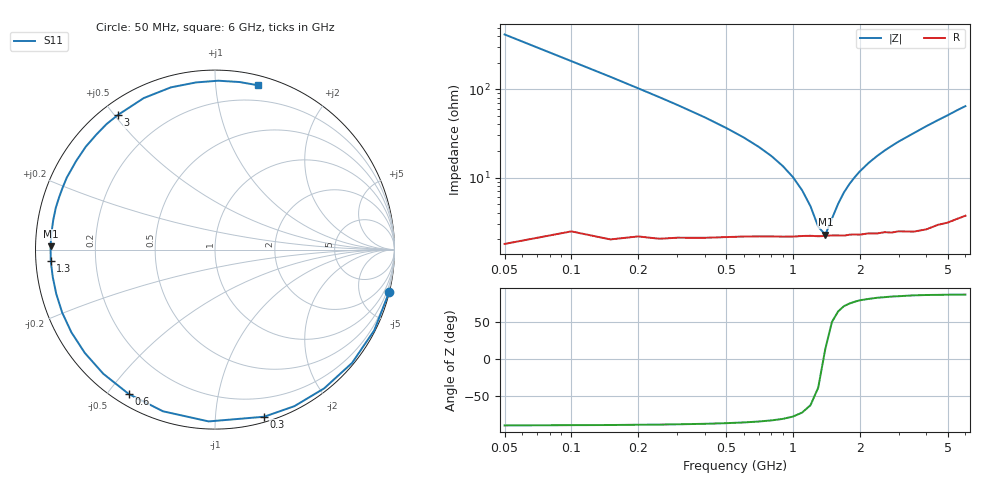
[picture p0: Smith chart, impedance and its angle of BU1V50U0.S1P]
! Infineon Technologies  Discrete & RF Semiconductors
! BB 833
! Si Tuning Diode in SOD323
! VR = 1.5 V
! S-Parameters:  June  1999
# GHz  S  MA  R  50
!  f  S11
! GHz  MAG  ANG
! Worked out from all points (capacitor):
!   34 points, 50 MHz to 6 GHz, reference 50 ohm
!   read as one part to ground: C = 7.57 pF near 50 MHz
!   lowest |Z| = 2.24 ohm at 1.4 GHz (marker M1)
!   series resonance near 1.377 GHz, so ESL is about 1.8 nH
!   S11 on the Smith chart (normalised r, x): 50 MHz: 0.04, -8.39; 300 MHz: 0.04, -1.34; 600 MHz: 0.04, -0.57; 1.3 GHz: 0.04, -0.03; 3 GHz: 0.05, +0.51; 6 GHz: 0.07, +1.29
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0.05  0.999 -13.6
0.1  0.9947 -26.9
0.15  0.9909 -39.6
0.2  0.9837 -51.8
0.25  0.9781 -63.1
0.3  0.9706 -73.6
0.4  0.9579 -92.1
0.5  0.9463 -107.8
0.6  0.9373 -120.8
0.7  0.9306 -132.0
0.8  0.9261 -141.6
0.9  0.9233 -150.1
1  0.9209 -157.6
1.1  0.9182 -164.4
1.3  0.9174 -176.0
1.4  0.9165 178.8
1.6  0.9162 169.6
1.8  0.9162 161.4
2  0.918 154.1
2.4  0.9204 141.5
2.8  0.9243 130.8
3  0.9249 125.9
3.5  0.9329 115.2
4  0.9368 105.2
4.5  0.9373 96.5
5  0.9412 88.9
5.5  0.9436 81.6
6  0.9462 75.5
